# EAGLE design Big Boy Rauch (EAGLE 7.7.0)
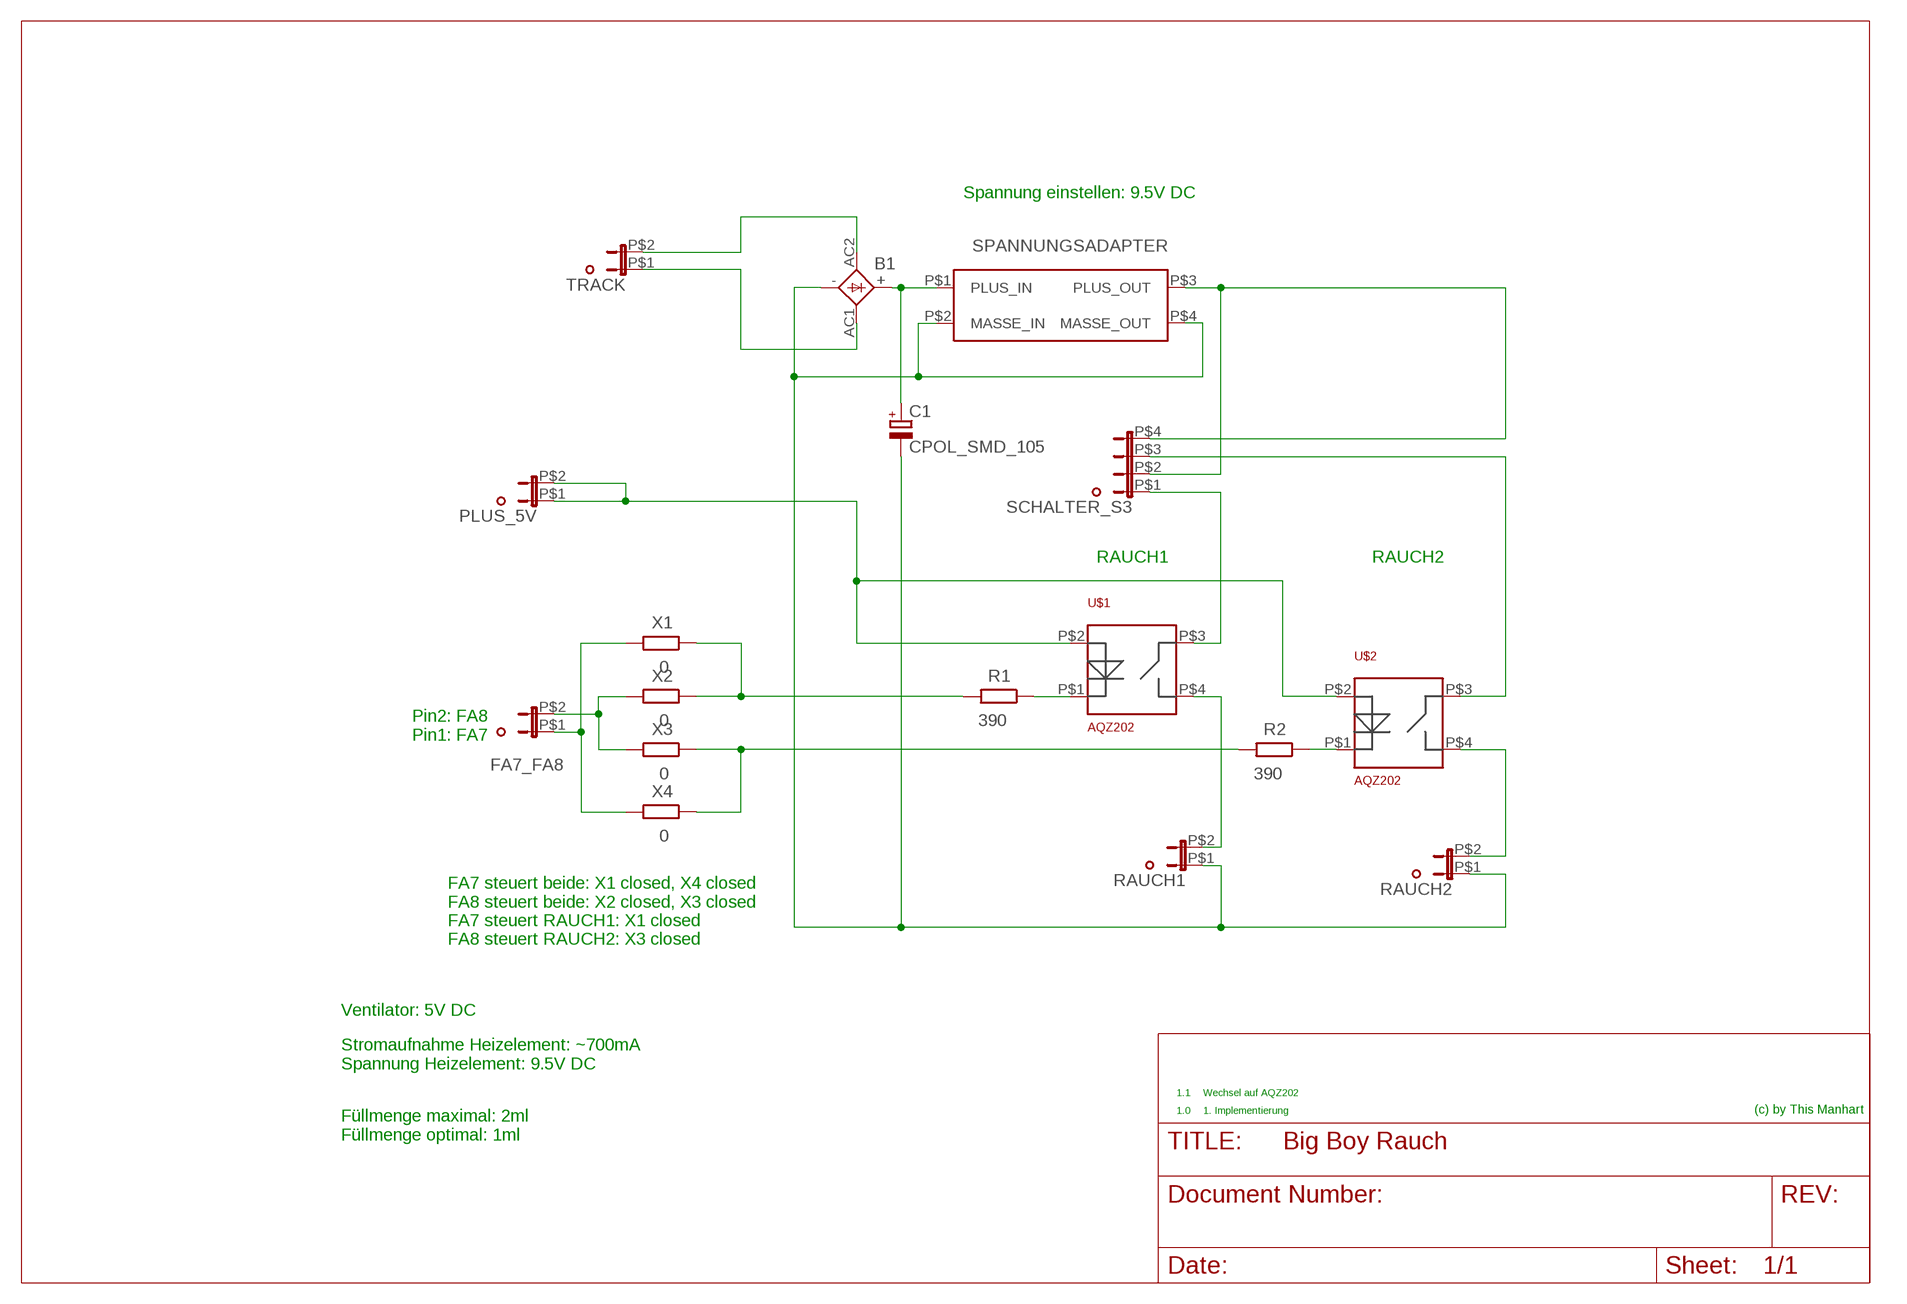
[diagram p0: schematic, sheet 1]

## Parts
B1  GBU4  [GBU4S]
C1  CPOL_SMD_105  [CPOL_SMD105_8X10.5]
FA7_FA8  DUBOX_2POL90  [DUBOX_2POL_STIFTLEISTE_90]
PLUS_5V  DUBOX_2POL90  [DUBOX_2POL_STIFTLEISTE_90]
R1  390  R-EU_R0805  [R0805]
R2  390  R-EU_R0805  [R0805]
RAUCH1  DUBOX_2POL90  [DUBOX_2POL_STIFTLEISTE_90]
RAUCH2  DUBOX_2POL90  [DUBOX_2POL_STIFTLEISTE_90]
SCHALTER_S3  DUBOX_4POL2REIHIG_90  [DUBOX_4POL_STIFTLEISTE_90_2R]
TRACK  DUBOX_2POL90  [DUBOX_2POL_STIFTLEISTE_90]
U$1  AQZ202  [AQZ202]
U$2  AQZ202  [AQZ202]
U$3  SPANNUNGSADAPTER  [SPANNUNGSADAPTER]
X1  0  R-EU_R0805  [R0805]
X2  0  R-EU_R0805  [R0805]
X3  0  R-EU_R0805  [R0805]
X4  0  R-EU_R0805  [R0805]

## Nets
N$1: B1.AC2(AC1) TRACK.P$2
N$2: B1.AC1(AC2) TRACK.P$1
N$3: RAUCH1.P$2 U$1.P$4(P3)
N$4: RAUCH2.P$2 U$2.P$4(P3)
N$5: PLUS_5V.P$1 PLUS_5V.P$2 U$1.P$2(P1) U$2.P$2(P1)
N$6: SCHALTER_S3.P$1 U$1.P$3(P4)
N$7: SCHALTER_S3.P$2 SCHALTER_S3.P$4 U$3.P$3(PLUS_OUT)
N$8: SCHALTER_S3.P$3 U$2.P$3(P4)
N$9: R1.1 U$1.P$1(P2)
N$10: R2.1 U$2.P$1(P2)
N$11: B1.+ C1.PLUS(+) U$3.P$1(PLUS_IN)
N$12: R2.2 X3.1 X4.1
N$13: R1.2 X1.1 X2.1
N$14: FA7_FA8.P$2 X2.2 X3.2
N$15: FA7_FA8.P$1 X1.2 X4.2
RAUCH2: B1.- C1.MINUS(-) RAUCH1.P$1 RAUCH2.P$1 U$3.P$2(MASSE_IN) U$3.P$4(MASSE_OUT)

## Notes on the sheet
- Spannung einstellen: 9.5V DC
- RAUCH1 | RAUCH2
- Pin2: FA8
  Pin1: FA7
- FA7 steuert beide: X1 closed, X4 closed
  FA8 steuert beide: X2 closed, X3 closed
  FA7 steuert RAUCH1: X1 closed
  FA8 steuert RAUCH2: X3 closed
- Ventilator: 5V DC
- Stromaufnahme Heizelement: ~700mA
  Spannung Heizelement: 9.5V DC
- 1.1 | Wechsel auf AQZ202
- 1.0 | 1. Implementierung | (c) by This Manhart
- Füllmenge maximal: 2ml
  Füllmenge optimal: 1ml

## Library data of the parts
B1 = rectifier:GBU4: GENERAL INSTRUMENT RECTIFIER
C1 = 0_mm:CPOL_SMD_105
FA7_FA8 PLUS_5V RAUCH1 RAUCH2 TRACK = 0_mm:DUBOX_2POL: DUBOX 2pol Buchse
R1 R2 X1-X4 = resistor:R-EU_: RESISTOR, European symbol
SCHALTER_S3 = 0_mm:DUBOX_4POL
U$1 U$2 = 0_mm:AQZ202
U$3 = 0_mm:SPANNUNGSADAPTER

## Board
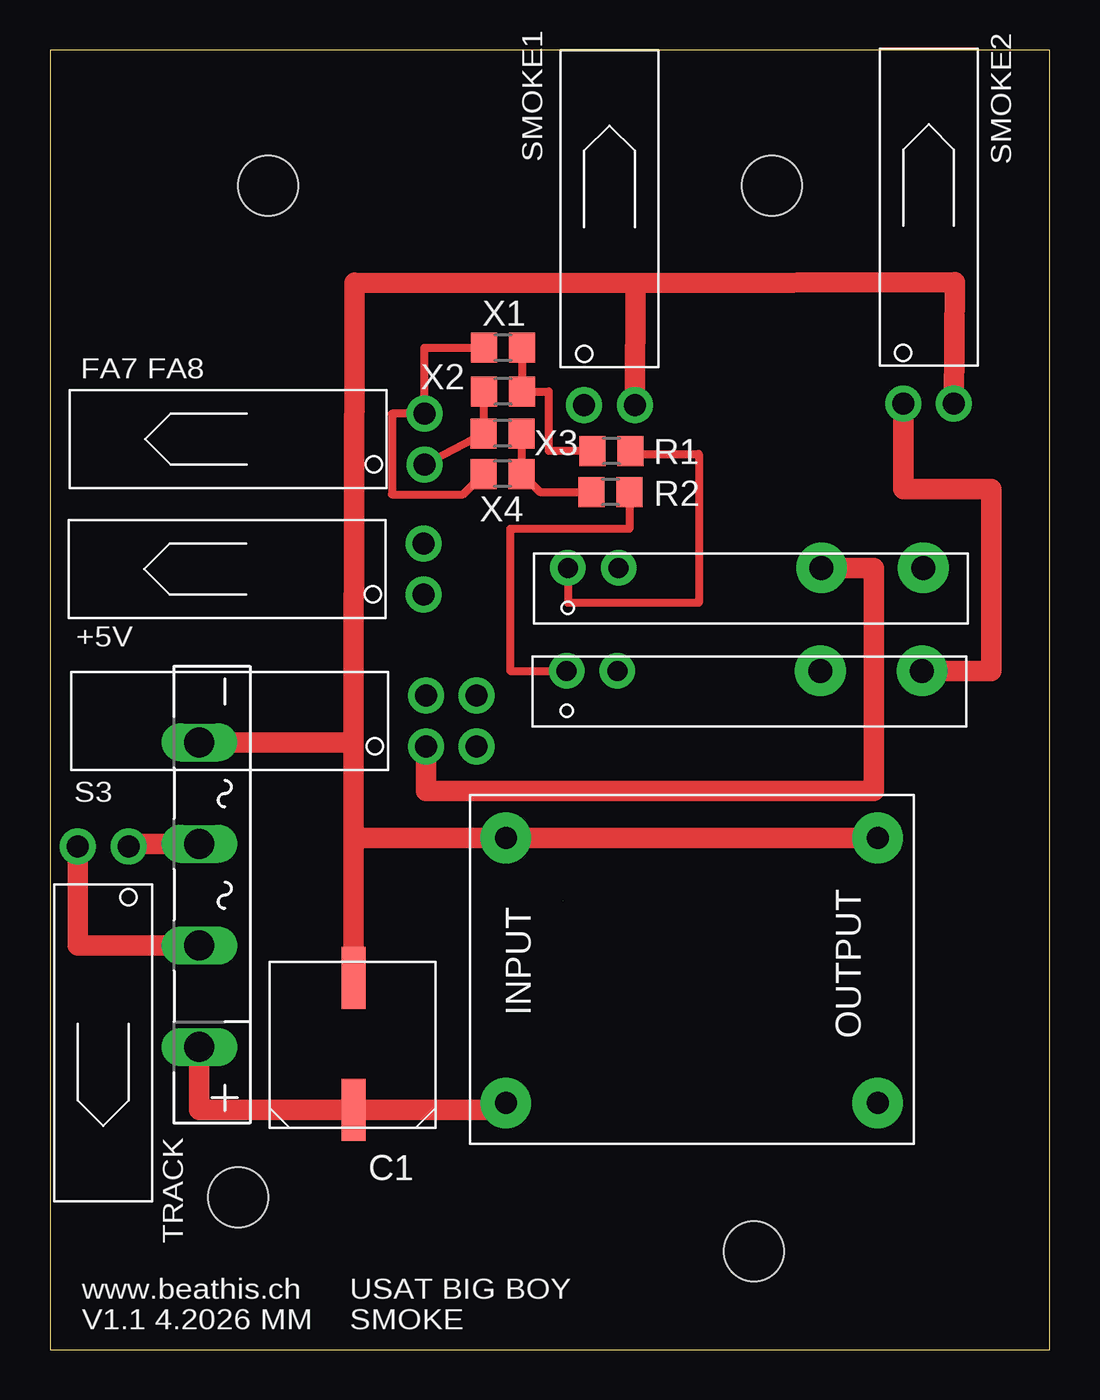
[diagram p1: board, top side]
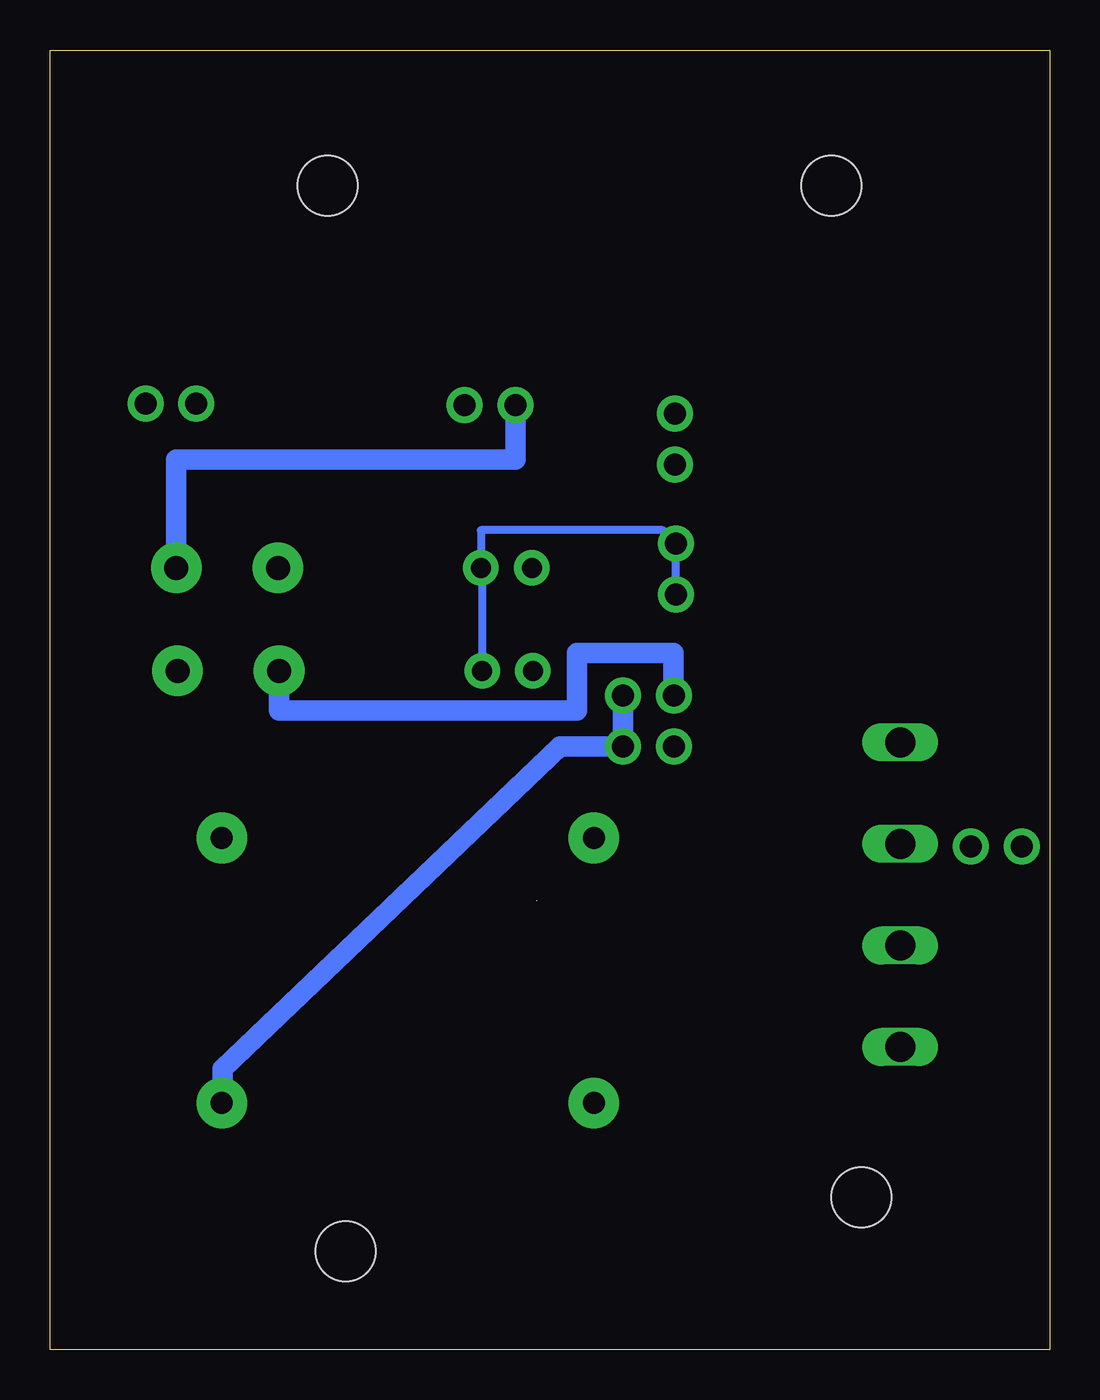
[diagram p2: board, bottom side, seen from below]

Size 50 x 65 mm. Coordinates in mm from the lower left corner, seen from the top.
Outline: 25.65,22.45 25.66,22.45
Outline: 50,0 50,65 0,65 0,0 50,0
Copper layers (1*16): Top 0.035mm / dielectric 1.5mm / Bottom 0.035mm
Design rules "PCB-POOL Standard": minimum track width 0.15mm, minimum drill 0.3mm, track to track 0.15mm, track to pad 0.15mm, pad to pad 0.15mm, via to via 0.15mm, smd to smd 0.15mm, copper to edge 0.3mm, drill to drill 0.2mm, minimum pad ring 0.2mm, minimum via ring 0.15mm, stop-mask expansion 0.075mm, vias tented up to drill 0mil, thermal gap 0.2mm
Holes 3 mm at 10.92,58.22 9.42,7.62 35.22,4.92 36.12,58.22

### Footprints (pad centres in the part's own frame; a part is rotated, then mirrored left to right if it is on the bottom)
GBU4S = drill 1.499 long: + 7.62,0; - -7.62,0; AC1 2.54,0; AC2 -2.54,0
CPOL_SMD105_8X10.5 = smd 1.2 x 3.1: MINUS 0,-3.5; PLUS 0,3.1
DUBOX_2POL_STIFTLEISTE_90 = drill 1.1 pad 1.8: P$1 1.27,0; P$2 -1.27,0
R0805 = smd 1.3 x 1.5: 1 -0.95,0; 2 0.95,0
DUBOX_4POL_STIFTLEISTE_90_2R = drill 1.1 pad 1.8: P$1 -1.27,0; P$2 -1.27,-2.54; P$3 1.27,0; P$4 1.27,-2.54
AQZ202 = drill 1 pad 1.778: P$1 0,0; P$2 2.54,0 | drill 1.2 pad 2.54: P$3 12.7,0; P$4 17.78,0
SPANNUNGSADAPTER = drill 1.1 pad 2.54: P$1 0,-13.26; P$2 0,0; P$3 18.6,-13.26; P$4 18.6,0

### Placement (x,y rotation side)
B1  7.47,22.75 270 top
C1  15.18,15.1 180 top
FA7_FA8  18.73,45.54 90 top
PLUS_5V  18.69,39.04 90 top
R1  28.08,44.94 180 top
R2  28.03,42.89 180 top
RAUCH1  27.99,47.25 0 top
RAUCH2  43.95,47.32 0 top
SCHALTER_S3  18.8,31.44 90 top
TRACK  2.66,25.17 180 top
U$1  25.9,39.1 0 top
U$2  25.84,33.95 0 top
U$3  22.8,25.59 0 top
X1  22.67,50.11 180 top
X2  22.67,47.92 180 top
X3  22.64,45.82 180 top
X4  22.64,43.8 180 top

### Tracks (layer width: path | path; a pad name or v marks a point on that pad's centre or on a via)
N$1
  Top 1.016: B1.AC2 3.93,25.29 TRACK.P$2
N$2
  Top 1.016: B1.AC1 1.39,20.21 TRACK.P$1
N$3
  Bottom 1.016: RAUCH1.P$2 26.72,44.51 43.69,44.51 U$1.P$4
N$4
  Top 1.016: RAUCH2.P$2 42.68,43.05 47.09,43.05 47.09,33.95 U$2.P$4
N$5
  Bottom 0.406: PLUS_5V.P$2 PLUS_5V.P$1 19.36,40.98 28.44,40.98 U$1.P$2 28.38,39.04 U$2.P$2
N$6
  Top 1.016: SCHALTER_S3.P$1 18.8,27.95 41.22,27.95 41.22,39.1 U$1.P$3
N$7
  Bottom 1.016: U$3.P$3 41.35,14.05 24.5,30.17 SCHALTER_S3.P$2 SCHALTER_S3.P$4
N$8
  Bottom 1.016: U$2.P$3 38.54,31.96 23.63,31.96 23.63,34.84 18.81,34.84 SCHALTER_S3.P$3
N$9
  Top 0.406: U$1.P$1 25.9,37.36 32.45,37.36 32.45,44.79 29.03,44.79 R1.1
N$10
  Top 0.406: R2.1 28.98,41.04 23.02,41.04 23.02,33.95 U$2.P$1
N$11
  Top 1.016: B1.+ 7.47,12 C1.PLUS 22.8,12 U$3.P$1
N$12
  Top 0.406: X3.1 X4.1 24.5,42.89 R2.2
N$13
  Top 0.406: X1.1 X2.1 24.94,47.92 24.94,44.96 27.13,44.96 R1.2
N$14
  Top 0.406: X2.2 21.69,47.92 X3.2 FA7_FA8.P$2
N$15
  Top 0.406: X1.2 18.73,50.11 FA7_FA8.P$1 17.1,46.81 17.1,42.77 20.66,42.77 X4.2
RAUCH2
  Top 1.016: B1.- 15.18,30.37 | 15.18,30.37 15.18,25.59 | 15.18,25.59 C1.MINUS | U$3.P$4 U$3.P$2 15.18,25.59 | 15.18,30.37 15.18,37.77 15.2,37.79 15.2,40.31 15.23,53.37 29.29,53.35 | 29.29,53.35 RAUCH1.P$1 | RAUCH2.P$1 45.27,53.4 29.29,53.35

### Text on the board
tNames: SMOKE1 | SMOKE2 | FA7 FA8 | +5V | S3 | TRACK | www.beathis.ch / V1.1 4.2026 MM | USAT BIG BOY / SMOKE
